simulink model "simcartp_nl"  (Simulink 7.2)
settings: Solver=ode45  StartTime=0.0  StopTime=500.0  RelTol=1e-3
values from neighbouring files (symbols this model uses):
  A = [0,1,0,0;0,0,-m/M*g,0;0,0,0,1;0,0,g/l*(M+m)/M,0]    [cartp.m]
  B = [0,0;1/M,-1/(l*M);0,0;-1/(M*l),1/l^2*(M+m)/(M*m)]    [cartp.m]
  C = [1,0,0,0;0,0,1,0]    [cartp.m]
  g = 9.8    [cartp.m]
  K = Ktot(1:4)    [cartp.m]
  ki = Ktot(5)    [cartp.m]
  l = 1    [cartp.m]
  L = -place(A',C(1,:)',roots(pobs))'    [cartp.m]
  m = 1    [cartp.m]
  M = 10    [cartp.m]
undefined symbols (not defined in the file or in its folder): Reference

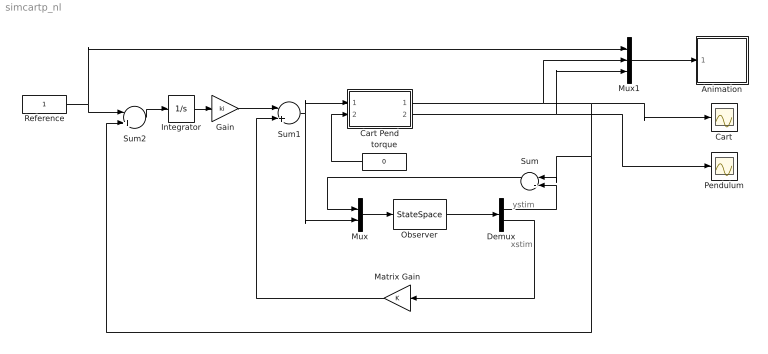
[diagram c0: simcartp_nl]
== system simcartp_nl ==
  note: xstim
  note: ystim
  Animation : Subsystem  mask(Pendulum plot){RefBlock=Reference}
      mask prompts: RefBlock "DC reference signal block name:"
      mask help: Pendulum plot
  Cart : Scope
  Cart Pend : Subsystem
  Demux : Demux  Outputs=[1;4]
  Gain : Gain  Gain=ki
  Integrator : Integrator
  Matrix Gain : Gain  Orientation=left  Gain=K  Multiplication=Matrix(K*u)
  Mux : Mux  Inputs=2
  Mux1 : Mux  Inputs=3
  Observer : StateSpace  A=A  B=[L,B(:,1)]  C=[C(1,:);eye(4)]  D=zeros(5,2)  X0=[0;0;0;0]
  Pendulum : Scope
  Reference : Constant
  Sum : Sum  Orientation=left  Inputs=|-|+
  Sum1 : Sum  Inputs=|++
  Sum2 : Sum  Inputs=|+-
  torque : Constant  Orientation=left  Value=0
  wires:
  Observer/1 -> Demux/1
  Demux/1 -> Sum/2
  Integrator/1 -> Gain/1
  Sum2/1 -> Integrator/1
  Mux/1 -> Observer/1
  Sum/1 -> Mux/1
  Gain/1 -> Sum1/1
  Sum1/1 -> Mux/2, Cart Pend/1(F)
  Reference/1 -> Sum2/1, Mux1/1
  Demux/2 -> Matrix Gain/1
  Matrix Gain/1 -> Sum1/2
  torque/1 -> Cart Pend/2(tau)
  Cart Pend/1(p) -> Sum2/2, Sum/1, Cart/1, Mux1/2
  Mux1/1 -> Animation/1(in_1)
  Cart Pend/2(theta) -> Pendulum/1, Mux1/3

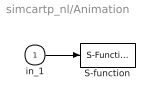
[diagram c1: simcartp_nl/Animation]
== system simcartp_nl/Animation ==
  in_1 : Inport
  S-function : S-Function  FunctionName=pendan  Parameters=RefBlock  EnableBusSupport=off
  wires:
  in_1/1 -> S-function/1

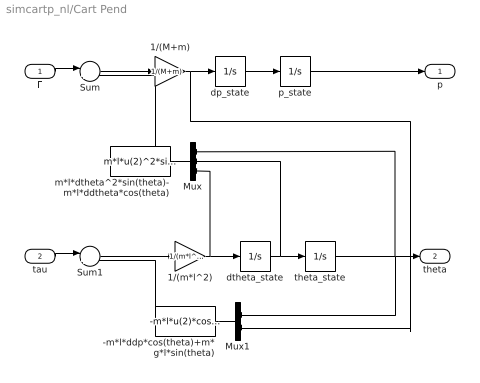
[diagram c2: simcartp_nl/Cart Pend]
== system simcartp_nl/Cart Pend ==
  F : Inport
  tau : Inport  Port=2
  -m*l*ddp*cos(theta)+m*g*l*sin(theta) : Fcn  Expr=-m*l*u(2)*cos(u(1))+m*g*l*sin(u(1))
  1/(M+m) : Gain  Gain=1/(M+m)
  1/(m*l^2) : Gain  Gain=1/(m*l^2)
  Mux : Mux  Inputs=3
  Mux1 : Mux  Inputs=2
  Sum : Sum  Inputs=|++
  Sum1 : Sum  Inputs=|++
  dp_state : Integrator
  dtheta_state : Integrator
  m*l*dtheta^2*sin(theta)-m*l*ddtheta*cos(theta) : Fcn  Expr=m*l*u(2)^2*sin(u(1))-m*l*u(3)*cos(u(1))
  p_state : Integrator
  theta_state : Integrator  InitialCondition=0.1
  p : Outport
  theta : Outport  Port=2
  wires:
  dp_state/1 -> p_state/1
  dtheta_state/1 -> theta_state/1, Mux/2
  1/(m*l^2)/1 -> dtheta_state/1, Mux/3
  Mux/1 -> m*l*dtheta^2*sin(theta)-m*l*ddtheta*cos(theta)/1
  theta_state/1 -> Mux/1, Mux1/1, theta/1
  Sum/1 -> 1/(M+m)/1
  m*l*dtheta^2*sin(theta)-m*l*ddtheta*cos(theta)/1 -> Sum/2
  -m*l*ddp*cos(theta)+m*g*l*sin(theta)/1 -> Sum1/2
  Mux1/1 -> -m*l*ddp*cos(theta)+m*g*l*sin(theta)/1
  1/(M+m)/1 -> Mux1/2, dp_state/1
  Sum1/1 -> 1/(m*l^2)/1
  F/1 -> Sum/1
  p_state/1 -> p/1
  tau/1 -> Sum1/1
